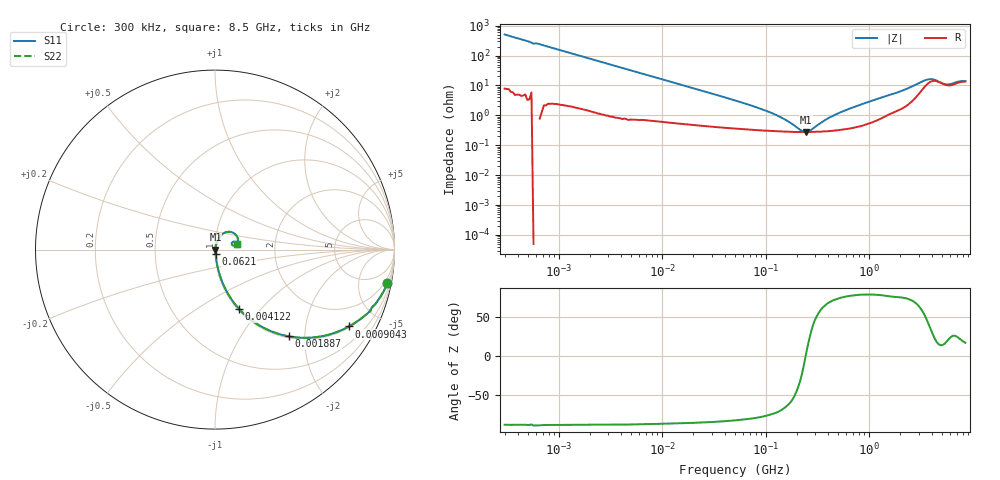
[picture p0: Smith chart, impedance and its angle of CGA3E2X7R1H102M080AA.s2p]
! S-parameter Generated by TDK Corporation
! Copyright(C) 2015 TDK Corporation.
! All Rights Reserved.
! TDK P/N: CGA3E2X7R1H102M080AA (Multilayer Ceramic Chip Capacitors)
! Property: C=1nF
! Size(LxWxT): 1.6x0.8x0.8mm, 0.063x0.031x0.031inches
! Model Type: s2p (Touchstone File Format Version 1.0)
! Frequency: DC=Yes Start=0.3MHz Stop=8500MHz 225points Log-sweep
! Note:
! Model Generated on Jun. 23, 2015
! Hash(MD5):
! Port Assignments:
!  1 ---| |--- 2
! Applicable Conditions:
!  Temperature = 25 degC
!  DC Bias Voltage = 0 V
!  Small Signal Operation
! Terms and conditions regarding TDK Simulation Models
! (1)This simulation model is being provided solely for informational purposes. Please refer to the specifications of the products in terms of detailed characteristics of such products.
! (2)In no event shall TDK Corporation of any of its subsidiaries be liable for any loss or damage arising, directly or indirectly,
!  From any information contained in this simulation model, including, but not limited to loss or damages arising from any inaccuracies, omissions or errors in connection with such information.
! (3)Any and all copyrights on this simulation model are owned by TDK Corporation.
!  Duplication or redistribution of this simulation model without prior written permission from TDK Corporation is prohibited.
! (4)This simulation model is subject to any modification or change without any prior notice.
! (5)Neither TDK Corporation nor any of its subsidiaries shall make any warranty, express or implied,
!  Including but not limited to the correctness, implied warranties of merchantability and fitness for a particular purpose with respect to this simulation models.
! (6)The use of this simulation model shall be deemed to have consented to the terms and conditions hereof.
# MHz S MA R 50
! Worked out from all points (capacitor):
!   224 points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, 300 kHz to 8.5 GHz, reference 50 ohm
!   read as one part in series: C = 1.05 nF near 314.1 kHz
!   lowest |Z| = 278 mohm at 246.6 MHz (marker M1)
!   series resonance near 243.4 MHz, so ESL is about 410 pH
!   S11 on the Smith chart (normalised r, x): 300 kHz: 1, -10; 904.3 kHz: 1.05, -3.46; 1.887 MHz: 1.03, -1.67; 4.122 MHz: 1.02, -0.77; 62.1 MHz: 1.01, -0.05; 8.5 GHz: 1.27, +0.08
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0.3  0.9783 -11.1  0.1927 78.0  0.1927 78.0  0.9783 -11.1
0.5710021  0.9278 -21.9  0.373 68.1  0.373 68.1  0.9278 -21.9
0.9042579  0.8606 -29.8  0.4975 59.4  0.4975 59.4  0.8606 -29.8
1.72111  0.6687 -47.1  0.7321 42.0  0.7321 42.0  0.6687 -47.1
1.88686  0.635 -49.6  0.7615 39.4  0.7615 39.4  0.635 -49.6
4.122422  0.3568 -68.0  0.9272 20.9  0.9272 20.9  0.3568 -68.0
9.430415  0.1663 -78.3  0.98 9.6  0.98 9.6  0.1663 -78.3
51.67171  0.03072 -81.6  0.996 1.7  0.996 1.7  0.03072 -81.6
62.1033  0.02524 -80.8  0.9963 1.4  0.9963 1.4  0.02524 -80.8
123.7646  0.01059 -73.4  0.997 0.6  0.997 0.6  0.01059 -73.4
163.0757  0.00644 -63.5  0.9971 0.3  0.9971 0.3  0.00644 -63.5
224.9819  0.002984 -22.3  0.9972 0.1  0.9972 0.1  0.002984 -22.3
246.6485  0.002772 4.0  0.9972 -0.0  0.9972 -0.0  0.002772 4.0
283.1228  0.003503 37.5  0.9972 -0.1  0.9972 -0.1  0.003503 37.5
373.0505  0.00687 64.6  0.9971 -0.4  0.9971 -0.4  0.00687 64.6
514.6664  0.01213 73.9  0.9967 -0.7  0.9967 -0.7  0.01213 73.9
1551.304  0.04688 74.4  0.9884 -2.6  0.9884 -2.6  0.04688 74.4
2572.272  0.08858 66.9  0.9686 -4.8  0.9686 -4.8  0.08858 66.9
3548.748  0.1383 42.5  0.9029 -5.9  0.9029 -5.9  0.1383 42.5
4073.536  0.141 25.3  0.8747 -4.0  0.8747 -4.0  0.141 25.3
5619.915  0.09773 16.9  0.9069 -1.8  0.9069 -1.8  0.09773 16.9
8500  0.1244 14.8  0.8803 -2.1  0.8803 -2.1  0.1244 14.8
